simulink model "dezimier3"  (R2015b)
settings: Solver=VariableStepAuto  StartTime=0.0  StopTime=10.0  RelTol=1e-3
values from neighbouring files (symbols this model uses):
  fst = 400    [dezimier_3.m]
  hanti = fir1(nord1, 1/M)    [dezimier_3.m]
  hTP = fir1(nord, 2*fp/fs)    [dezimier_2.m]    (also in dezimier_3.m; frac_delay_1.m = fir1(nord, fp*2); frac_delay_2.m = fir1(nord, fp*2); lagrange_3.m = fir1(40, 0.5))
  M = 5    [dezimier_1.m]    (also in dezimier_11.m; dezimier_2.m; dezimier_3.m; farrow_3.m)
  nord1 = 256    [basisband_2.m]    (also in dezimier_3.m; poly_dez_1.m = 32; poly_dez_2.m = 32; poly_interp_1.m = 32)
  Ts = 1/fs    (= 5e-05)    [basisband_1.m]    (also in basisband_2.m = 5e-06; dezimier_1.m = 0.0005; dezimier_11.m = 0.0005; dezimier_2.m = 0.0005)
libraries: simulink x1, dspsigops x1

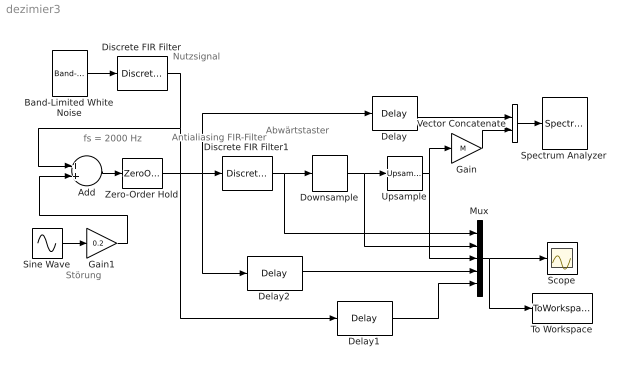
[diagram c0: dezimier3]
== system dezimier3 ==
  note: Nutzsignal
  note: Antialiasing FIR-Filter
  note: Störung
  note: Abwärtstaster
  note: fs = 2000 Hz
  Add : Sum
  Band-Limited White Noise : simulink/Sources/Band-Limited White Noise  Cov=Ts/10  Ts=Ts  seed=[23341]
  Delay : Delay  DelayLength=nord1/2
  Delay1 : Delay  DelayLength=nord1/2
  Delay2 : Delay  DelayLength=nord1/2
  Discrete FIR Filter1 : DiscreteFir  Coefficients=hanti  SampleTime=Ts
  Discrete FIR Filter : DiscreteFir  Coefficients=hTP  SampleTime=Ts
  Downsample : DownSample  N=M  RateOptions=Allow multirate processing
  Gain : Gain  Gain=M
  Gain1 : Gain  Gain=0.2
  Mux : Mux  Inputs=5
  Scope : Scope
  Sine Wave : Sin  Frequency=2*pi*fst  SampleTime=Ts
  Spectrum Analyzer : SpectrumAnalyzer
  To Workspace : ToWorkspace  VariableName=y  SaveFormat=Timeseries  SampleTime=-1
  Upsample : dspsigops/Upsample  N=M  phase=0  RateOptions=Allow multirate processing  ic=0  mode=Unused parameter value
  Vector Concatenate : Concatenate  Mode=Multidimensional array  ConcatenateDimension=2
  Zero-Order Hold : ZeroOrderHold  SampleTime=Ts
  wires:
  Mux/1 -> To Workspace/1, Scope/1
  Zero-Order Hold/1 -> Delay/1, Delay2/1, Discrete FIR Filter1/1
  Vector Concatenate/1 -> Spectrum Analyzer/1
  Band-Limited White Noise/1 -> Discrete FIR Filter/1
  Upsample/1 -> Gain/1, Mux/3
  Gain/1 -> Vector Concatenate/2
  Add/1 -> Zero-Order Hold/1
  Discrete FIR Filter/1 -> Delay1/1, Add/1
  Sine Wave/1 -> Gain1/1
  Delay/1 -> Vector Concatenate/1
  Downsample/1 -> Mux/2, Upsample/1
  Gain1/1 -> Add/2
  Delay2/1 -> Mux/4
  Discrete FIR Filter1/1 -> Mux/1, Downsample/1
  Delay1/1 -> Mux/5
